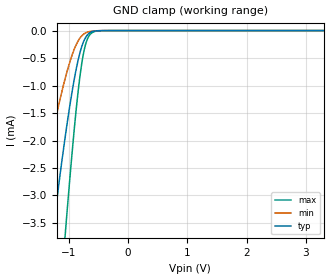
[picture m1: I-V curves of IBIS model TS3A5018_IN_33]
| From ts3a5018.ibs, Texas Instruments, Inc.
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[Model]   TS3A5018_IN_33
Model_type  Input
Vinl=0.8
Vinh=2.0
| variable   typ   min   max
C_comp   2.42pF   1.60pF   2.83pF
[Temperature Range]   40   100   -40
| Ambient temperature   25   85   -40
[Voltage range]   3.3   3   3.6
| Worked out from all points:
|   GND clamp passes 1 mA (typ) near -0.93 V on its own axis
[GND Clamp]
| TS3A5018_IN_33
|   Voltage   I(typ)   I(min)   I(max)
-3.3V     -29.67mA   -19.35mA   -43.12mA
-1.585V   -6.868mA   -3.788mA   -11.62mA
-1.545V   -6.434mA   -3.518mA   -10.97mA
-1.265V   -3.652mA   -1.837mA   -6.602mA
-1.065V   -1.972mA   -889.7uA   -3.78mA
-1.035V   -1.746mA   -769.1uA   -3.381mA
-850mV    -574.9uA   -204.3uA   -1.184mA
-785mV    -305.3uA   -101.1uA   -628.5uA
-720mV    -134.3uA   -45.52uA   -266uA
-625mV    -28.19uA   -13.63uA   -53.71uA
-435mV    -753.9nA   -328.2nA   -1.808uA
3.3V      128.2pA    10.12pA    1.439nA
